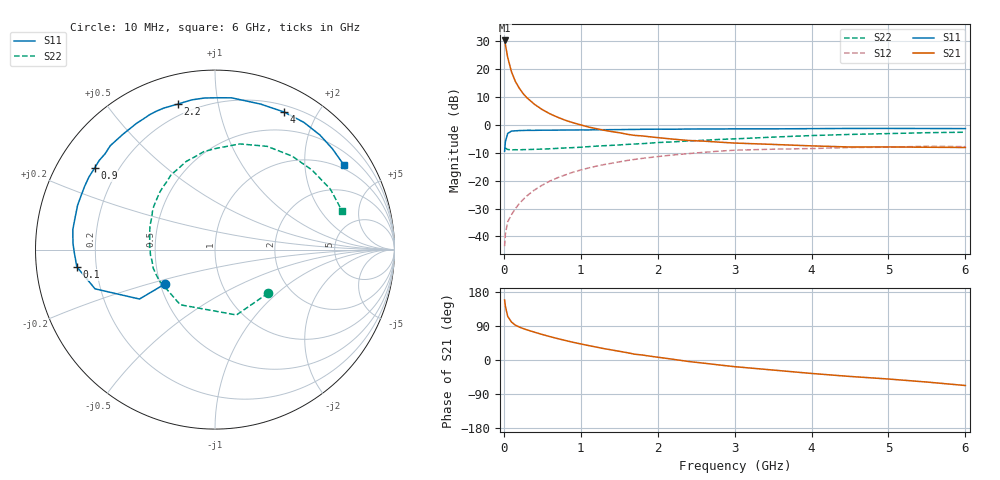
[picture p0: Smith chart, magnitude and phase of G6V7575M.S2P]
! SIEMENS Small Signal Semiconductors
! BFG193
! Si NPN RF Bipolar Junction Transistor in SOT223
! VCE = 0.75 V  IC = 75 mA
! Common Emitter S-Parameters:  August  1996
# GHz  S  MA  R  50
!  f  S11  S21  S12  S22
! GHz  MAG  ANG  MAG  ANG  MAG  ANG  MAG  ANG
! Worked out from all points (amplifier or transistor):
!   36 points, 10 MHz to 6 GHz, reference 50 ohm
!   highest |S21| = 30.3 dB at 10 MHz (marker M1)
!   |S21| within 3 dB of that: start of sweep to 30.09 MHz
!   unconditionally stable (mu >= 1): start of sweep to 30.1 MHz; 90.3 MHz to end of sweep
!   at 250 MHz: K = 1.27, MAG = 15.9 dB, |S12| = -26.8 dB
!   at 1.4 GHz: K = 1.26, MAG = 2.6 dB, |S12| = -13.8 dB
!   at 6 GHz: K = 1.08, MAG = -1.9 dB, |S12| = -7.8 dB
!   S11 on the Smith chart (normalised r, x): 10 MHz: 0.53, -0.23; 100 MHz: 0.13, -0.06; 900 MHz: 0.11, +0.30; 2.2 GHz: 0.14, +0.77; 4 GHz: 0.27, +1.59; 6 GHz: 0.87, +3.12
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0.01  0.3373 -145.5  32.69 158.5  0.0067 61.7  0.3827 -39.3
0.02  0.5029 -146.8  27.69 142.1  0.0111 56.4  0.3833 -71.8
0.05  0.7033 -161.9  16.25 115.3  0.0183 47.5  0.3633 -122.2
0.1  0.7758 -172.9  8.906 100.0  0.0247 52.3  0.3562 -151.5
0.15  0.7839 -178.7  6.021 92.0  0.0315 56.1  0.3597 -163.3
0.2  0.7918 177.6  4.57 87.1  0.0388 60.2  0.3564 -169.6
0.25  0.7953 174.7  3.656 83.0  0.0459 62.0  0.3609 -175.0
0.3  0.7999 171.9  3.07 79.6  0.0535 63.2  0.3609 -178.1
0.4  0.7997 167.0  2.332 73.3  0.0684 63.6  0.3652 175.6
0.5  0.8044 162.2  1.881 67.3  0.0832 62.6  0.3686 170.7
0.6  0.8044 158.0  1.58 61.7  0.0987 61.3  0.3734 166.7
0.7  0.8073 154.2  1.372 56.4  0.1132 59.6  0.38 162.9
0.9  0.8104 145.9  1.094 46.7  0.1422 54.9  0.3918 155.1
1.1  0.8124 139.0  0.917 38.1  0.169 50.3  0.4076 148.8
1.7  0.83 118.9  0.649 15.3  0.2408 34.6  0.4548 129.1
2.2  0.8368 104.4  0.556 1.9  0.2893 20.8  0.496 114.2
2.8  0.8463 88.4  0.491 -13.1  0.3392 5.1  0.5493 96.5
3.5  0.8497 72.6  0.447 -26.5  0.3671 -13.4  0.6048 76.8
4  0.8576 63.4  0.421 -35.5  0.377 -23.0  0.6446 63.2
4.5  0.8647 55.1  0.402 -43.4  0.3939 -32.5  0.6752 50.5
5.5  0.8622 40.6  0.398 -58.2  0.4144 -53.8  0.7256 27.7
6  0.859 33.3  0.394 -67.3  0.4082 -65.8  0.7398 17.0
